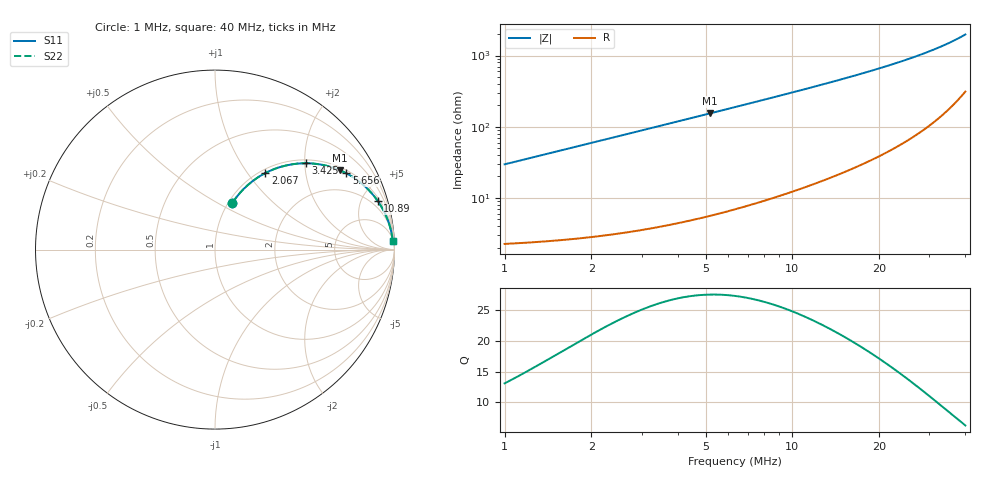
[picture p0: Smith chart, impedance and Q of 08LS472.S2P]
! Coilcraft 0805LS-472 Chip Inductor
! 18 September 2002
# MHZ S MA R 50
!Freq  MagS11  AngS11  MagS21  AngS21  MagS12  AngS12  MagS22  AngS22
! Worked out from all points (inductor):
!   404 points, 1 MHz to 40 MHz, reference 50 ohm
!   read as one part in series: L = 4.7 uH near 1.194 MHz
!   highest Q = 27.5 at 5.171 MHz (marker M1), where L = 4.73 uH
!   S11 on the Smith chart (normalised r, x): 1 MHz: 1.05, +0.59; 2.067 MHz: 1.06, +1.22; 3.425 MHz: 1.08, +2.03; 5.656 MHz: 1.12, +3.37; 10.89 MHz: 1.28, +6.63; 40 MHz: 7, +39
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1  0.2783 69.5  0.9395 -16.1  0.9395 -16.1  0.2783 69.5
1.194  0.3265 67.2  0.9238 -19.0  0.9238 -19.0  0.3265 67.2
1.388  0.3722 64.8  0.9062 -21.8  0.9062 -21.8  0.3722 64.8
1.582  0.4153 62.4  0.8873 -24.5  0.8873 -24.5  0.4153 62.4
1.776  0.4557 60.0  0.8673 -27.1  0.8673 -27.1  0.4557 60.0
2.067  0.5112 56.6  0.8359 -30.7  0.8359 -30.7  0.5112 56.6
2.649  0.605 50.4  0.7715 -37.2  0.7715 -37.2  0.605 50.4
3.037  0.6559 46.8  0.7293 -40.9  0.7293 -40.9  0.6559 46.8
3.425  0.699 43.5  0.6888 -44.3  0.6888 -44.3  0.699 43.5
4.298  0.7733 37.3  0.6062 -50.6  0.6062 -50.6  0.7733 37.3
5.171  0.8248 32.4  0.5363 -55.5  0.5363 -55.5  0.8248 32.4
5.656  0.8465 30.1  0.5026 -57.8  0.5026 -57.8  0.8465 30.1
6.529  0.8768 26.7  0.4498 -61.2  0.4498 -61.2  0.8768 26.7
7.596  0.9032 23.4  0.3967 -64.5  0.3967 -64.5  0.9032 23.4
9.051  0.9273 19.8  0.3397 -67.9  0.3397 -67.9  0.9273 19.8
10.894  0.9467 16.6  0.2854 -71.1  0.2854 -71.1  0.9467 16.6
14.095  0.9653 12.7  0.2202 -74.6  0.2202 -74.6  0.9653 12.7
17.102  0.9747 10.3  0.1786 -76.7  0.1786 -76.7  0.9747 10.3
20.594  0.9811 8.3  0.1439 -78.3  0.1439 -78.3  0.9811 8.3
27.093  0.9871 5.7  0.1003 -79.7  0.1003 -79.7  0.9871 5.7
33.592  0.9898 4.1  0.07123 -79.7  0.07123 -79.7  0.9898 4.1
40  0.9909 2.8  0.05004 -78.1  0.05004 -78.1  0.9909 2.8
